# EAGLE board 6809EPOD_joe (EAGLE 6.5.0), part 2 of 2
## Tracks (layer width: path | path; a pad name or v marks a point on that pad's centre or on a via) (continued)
N$122  (via drill 0.2) (continued)
  Top 0.152: v44.73,49.61 44.27,50.06 40.92,50.06 40.16,50.82 32.54,50.82 31.62,51.74 18.21,51.74 17.91,51.44 17.91,50.52 17.45,50.06 12.57,50.06 12.27,49.76 12.27,49.15 v11.66,48.54
  Bottom 0.152: U14.5 47.07,46.96 45.19,46.96 44.73,47.47 v44.73,49.61 | RS11.R4A 10.36,49 11.2,49 v11.66,48.54
N$123  (via drill 0.2)
  Top 0.152: v45.03,50.82 44.58,50.37 41.07,50.37 40.31,51.13 32.69,51.13 31.77,52.05 18.06,52.05 17.6,51.59 17.6,50.67 17.3,50.37 12.12,50.37 v11.51,49.76
  Bottom 0.152: 47.07,49.5 U14.7 47.07,49.55 45.8,49.55 45.49,49.86 45.49,50.37 v45.03,50.82 | RS11.R3A v11.51,49.76
N$124  (via drill 0.2)
  Top 0.152: U5.14 19.3,9.37 20.8,9.37 21.72,8.46 23.7,8.46 24.15,8 28.27,8 29.79,6.48 36.04,6.48 37.57,4.95 38.33,4.95 38.79,5.41 38.79,7.24 39.55,8 39.55,9.22 40.92,10.59 40.92,11.2 41.53,11.81 46.41,11.81 v47.02,12.42 | v49.61,27.51 v51.89,27.51
  Bottom 0.152: v47.02,12.42 47.02,13.49 49.61,16.08 49.61,19.89 49,20.5 49,21.41 49.61,22.02 v49.61,27.51 | v51.89,27.51 54.33,27.51 54.79,27.96 54.79,30.71 54.48,31.01 52.65,31.01 53.42,31.17 53.37,31.12 U2.12
N$125  (via drill 0.2)
  Top 0.152: v17.45,16.84 17.75,17.14 U5.8 19.13,17.14
  Bottom 0.152: U10.3 17.6,20.95 17.45,20.8 17.45,19.74 | v17.45,16.84 17.45,19.74 | U10.2 19.1,19.74 17.45,19.74
N$126  (via drill 0.2)
  Top 0.152: v17.45,22.17 18.06,21.56 20.8,21.56 22.02,22.78 v33.15,22.78 | U6.6 37.01,34.87 36.96,34.98 34.82,34.98 v33.76,33.91
  Bottom 0.152: U10.4 19.07,22.22 18.82,22.17 v17.45,22.17 | v33.15,22.78 33.76,23.39 v33.76,33.91
N$127
  Top 0.152: U5.13 19.1,10.74 17.91,10.74 17.6,11.05 17.6,14.25 17.91,14.55 19.05,14.55 U5.10
N$128  (via drill 0.2)
  Top 0.152: v20.8,24.92 21.72,24.92 22.63,24 28.42,24 v28.88,24.46
  Bottom 0.152: U10.6 19.15,24.74 19.28,24.92 v20.8,24.92 | v28.88,24.46 28.88,23.85 29.18,23.55 30.56,23.55 30.58,23.52 U9.5
N$129  (via drill 0.2)
  Top 0.152: v22.78,16.99 24.92,16.99 25.07,17.14 U5.7 | U5.12 19.2,12.12 v22.33,12.12 | v29.03,21.56 28.12,22.48 24.92,22.48 24,21.56 23.39,21.56 v22.48,20.65
  Bottom 0.152: 25.68,19.74 25.63,19.68 U10.13 25.25,19.89 22.48,19.89 | 22.48,19.89 22.78,19.58 v22.78,16.99 22.33,16.69 v22.33,12.12 | U9.4 30.2,22.38 30.15,22.22 30,22.22 30.1,22.33 29.18,22.33 29.03,22.17 v29.03,21.56 | 22.48,19.89 v22.48,20.65
N$130  (via drill 0.2)
  Top 0.152: v23.7,20.8 24.46,20.8 24.61,20.65 27.81,20.65 v28.88,19.58
  Bottom 0.152: v23.7,20.8 25.22,20.8 25.07,20.95 U10.12 | U9.2 30.53,19.58 v28.88,19.58 28.88,18.82 29.18,18.52 30.48,18.52 U9.1
N$131  (via drill 0.2)
  Top 0.152: v33.15,9.07 33.15,9.98 34.82,11.66 34.82,13.03 35.13,13.34 U7.4 | v33.15,21.41 v33.15,19.43
  Bottom 0.152: v33.15,19.43 31.77,20.8 31.01,20.8 30.4,20.95 U9.3 | v33.15,9.07 32.69,9.53 32.69,12.57 34.21,14.1 34.21,15.32 33.3,16.23 33.3,16.99 34.37,18.06 34.37,20.19 v33.15,21.41
N$132  (via drill 0.2)
  Top 0.152: U5.3 25.3,11.96 v27.05,11.96 | U7.6 36.7,15.88 36.65,15.77 35.28,15.77 34.21,14.71 v33.3,14.71
  Bottom 0.152: v27.05,11.96 27.66,12.57 27.66,16.38 28.27,16.99 30.1,16.99 32.38,14.71 v33.3,14.71
RS17_TGT_BA  (via drill 0.2)
  Top 0.152: v73.23,4.65 73.23,6.17 73.53,6.48 79.17,6.48 79.78,7.09 v84.05,7.09
  Bottom 0.152: U13_PIGGY.3 71.55,5.71 71.7,5.56 72.92,5.56 73.23,5.26 v73.23,4.65 | v84.05,7.09 84.35,7.39 84.35,14.71 TGT_HDR.6
RS17_TGT_BS  (via drill 0.2)
  Top 0.152: v72.47,11.96 72.47,11.51 72.77,11.2 77.19,11.2 77.95,11.96 81.76,11.96 83.13,13.34 TGT_HDR.5
  Bottom 0.152: U13_PIGGY.6 72.47,9.53 72.62,9.68 72.62,11.81 v72.47,11.96
SEL_ADDR_TO_TGT  (via drill 0.2)
  Top 0.152: J8.11 5.82,15.88 5.87,15.93 9.07,15.93 10.13,16.99 16.54,16.99 17.91,18.36 v21.41,18.36 | U3.6 25.22,34.21 v23.7,34.21
  Bottom 0.152: v21.41,18.36 20.65,19.13 20.65,21.56 22.33,23.24 22.33,25.38 24.92,27.96 24.92,33.6 24.31,34.21 v23.7,34.21
SEL_ADDR_TO_TGT'  (via drill 0.2)
  Top 0.152: U20.1 67.74,41.88 v67.74,40.62 | v66.98,29.18 66.37,29.79 66.37,34.67 v66.83,35.13 | U22.1 68.5,2.51 66.83,2.51 66.52,2.82 v66.52,3.43 | 25.32,35.59 25.38,35.59 | 25.32,35.59 U3.7 | v51.28,35.59 55.7,35.59 56.46,34.82 59.36,34.82 59.82,34.37 v60.43,34.37 | U7.12 30.63,12.12 | v45.49,16.84 44.88,16.84 44.58,17.14 39.7,17.14 39.24,17.6 39.24,18.67 38.79,19.13 36.5,19.13 35.28,17.91 35.28,16.54 34.21,15.47 32.84,15.47 32.54,15.16 32.54,14.25 32.23,13.95 29.03,13.95 28.73,13.64 28.73,12.12 | v49,17.6 50.52,17.6 50.82,17.3 50.82,14.71 51.13,14.4 52.65,14.4 53.57,15.32 55.4,15.32 55.7,15.62 55.7,16.38 56.62,17.3 58.75,17.3 59.82,18.36 59.82,19.89 60.27,20.34 64.24,20.34 65.15,21.26 66.22,21.26 66.67,21.72 v66.67,23.09 | 25.32,35.59 24,35.59 v23.39,36.2 22.48,35.28 22.48,27.81 23.39,26.9 27.05,26.9 v28.27,25.68 | v27.2,10.9 27.66,10.9 27.96,11.2 27.96,11.81 28.27,12.12 28.73,12.12 | U7.12 30.45,12.07 30.4,12.12 28.73,12.12 | 30.71,12.12 30.66,12.07 U7.12
  Bottom 0.152: U19.1 71.25,40.62 v67.74,40.62 66.83,39.7 v66.83,35.13 61.19,35.13 v60.43,34.37 | U21.1 69.93,29.18 v66.98,29.18 66.98,28.12 67.59,27.51 67.59,23.09 | 67.59,23.09 67.59,21.26 67.89,20.95 67.89,15.01 67.28,14.4 67.28,11.35 65.61,9.68 65.61,8.31 66.06,7.85 66.06,3.89 v66.52,3.43 | U13.11 23.7,47.62 23.24,47.17 23.24,41.99 24.31,40.92 24.31,37.11 v23.39,36.2 | U2.10 53.14,33.6 52.05,33.6 51.28,34.37 v51.28,35.59 | v45.49,16.84 45.8,17.14 U8.2 48.54,17.14 v49,17.6 | v66.67,23.09 67.59,23.09 | v28.27,25.68 28.27,19.89 27.96,19.58 27.96,17.91 25.53,15.47 25.53,11.51 26.14,10.9 v27.2,10.9
TGT_A0  (via drill 0.2)
  Top 0.152: TGT_HDR.8 81.81,19.58 79.02,19.58 77.34,21.26 v74.3,21.26 | U22.4 68.5,6.33 72.47,6.33 73.53,7.39 v73.99,7.39
  Bottom 0.152: v73.99,7.39 74.45,7.85 74.45,9.83 73.99,10.29 73.99,15.93 74.3,16.23 v74.3,21.26
TGT_A1  (via drill 0.2)
  Top 0.152: TGT_HDR.9 81.86,22.17 81.86,20.45 81.3,19.89 79.17,19.89 76.89,22.17 v74.3,22.17 | U22.7 68.5,10.13 69.88,10.13 70.03,9.98 70.03,8 70.48,7.54 72.92,7.54 v73.69,8.31
  Bottom 0.152: v73.69,8.31 74.14,8.76 74.14,9.68 73.69,10.13 73.69,16.08 73.99,16.38 73.99,20.65 73.69,20.95 73.69,21.56 v74.3,22.17
TGT_A2  (via drill 0.2)
  Top 0.152: v78.56,24.61 77.8,25.38 76.73,25.38 76.12,24.77 71.25,24.77 69.88,26.14 v65.15,26.14 | U22.9 62.41,11.35 v64.08,11.35
  Bottom 0.152: TGT_HDR.10 81.76,24.61 v78.56,24.61 | v64.08,11.35 65.15,11.35 65.46,11.66 65.46,12.57 65.15,12.88 65.15,15.32 65.46,15.62 65.46,18.82 65.91,19.28 65.91,21.11 65.15,21.87 v65.15,26.14
TGT_A3  (via drill 0.2)
  Top 0.152: v66.83,27.2 67.59,26.44 70.03,26.44 71.4,25.07 75.97,25.07 77.19,26.29 v77.95,26.29 | U22.12 62.41,7.54 v64.69,7.54
  Bottom 0.152: v64.69,7.54 64.69,10.13 65.76,11.2 65.76,12.73 65.46,13.03 65.46,15.16 65.76,15.47 65.76,18.67 66.22,19.13 66.22,21.26 65.46,22.02 65.46,23.55 65.76,23.85 66.83,23.85 67.28,24.31 67.28,26.75 v66.83,27.2 | v77.95,26.29 79.48,27.51 82.07,27.51 83.13,28.57 TGT_HDR.11
TGT_A4  (via drill 0.2)
  Top 0.152: TGT_HDR.12 83.13,31.17 82.07,30.1 82.07,25.07 81.61,24.61 79.93,24.61 78.72,25.83 78.72,26.59 78.26,27.05 71.7,27.05 71.25,26.59 70.33,26.59 v69.72,27.2
  Bottom 0.152: U21.4 69.98,32.99 71.25,32.99 71.55,32.69 71.55,28.57 71.25,28.27 70.18,28.27 69.72,27.81 v69.72,27.2
TGT_A5  (via drill 0.2)
  Top 0.152: TGT_HDR.13 81.76,32.23 81.76,25.22 81.46,24.92 80.09,24.92 79.02,25.98 79.02,26.75 78.41,27.36 v70.79,27.36
  Bottom 0.152: U21.7 69.98,36.8 71.55,36.8 71.86,36.5 71.86,28.42 v70.79,27.36
TGT_A6  (via drill 0.2)
  Top 0.152: v78.26,37.57 81.91,37.57 83.13,36.35 83.13,36.25 TGT_HDR.14
  Bottom 0.152: U21.9 76.17,38.18 77.65,38.18 v78.26,37.57
TGT_A7
  Bottom 0.152: U21.12 75.87,34.06 78.56,34.06 79.48,34.98 79.48,37.11 79.93,37.57 81.91,37.57 83.13,38.79 TGT_HDR.15
TGT_A8
  Top 0.152: U20.4 68.55,45.8 76.28,45.8 77.04,45.03 81.46,45.03 81.91,44.58 81.91,42.6 83.13,41.38 83.13,41.33 TGT_HDR.16
TGT_A9  (via drill 0.2)
  Top 0.152: U20.7 68.5,49.55 68.5,49.61 69.88,49.61 70.33,49.15 70.33,46.56 70.79,46.1 77.95,46.1 v79.32,47.47
  Bottom 0.152: TGT_HDR.17 81.91,45.09 81.91,46.86 81.3,47.47 v79.32,47.47
TGT_A10
  Top 0.152: TGT_HDR.18 81.91,47.62 80.24,47.62 78.41,49.45 73.23,49.45 71.25,51.44 65.76,51.44 65,50.67 62.36,50.67 U20.9
TGT_A11  (via drill 0.2)
  Top 0.152: TGT_HDR.19 82.02,50.06 79.93,50.06 78.87,51.13 72.92,51.13 v72.62,51.44 | U20.12 62.36,47.02 v64.54,47.02
  Bottom 0.152: v64.54,47.02 60.58,47.02 60.27,47.32 60.27,50.06 61.65,51.44 v72.62,51.44
TGT_A12
  Bottom 0.152: U19.4 71.25,44.42 73.38,44.42 73.99,45.03 73.99,48.39 73.53,48.84 73.53,50.67 73.99,51.13 78.87,51.13 79.78,50.22 82.07,50.22 83.13,51.28 83.13,51.44 TGT_HDR.20
TGT_A13
  Bottom 0.152: U19.7 71.25,48.23 72.62,48.23 73.23,48.84 73.23,50.82 73.84,51.44 TGT_HDR.21
TGT_A14
  Bottom 0.152: U19.9 77.44,49.61 78.87,49.61 79.63,48.84 80.7,48.84 TGT_HDR.22
TGT_A15
  Bottom 0.152: U19.12 77.44,45.8 78.87,45.8 79.48,46.41 80.59,46.41 TGT_HDR.23
TGT_AVMA  (via drill 0.2)
  Top 0.152: v73.08,19.13 78.11,19.13 79.93,17.3 81.3,17.3 81.76,16.84 81.76,14.4 80.7,13.34 80.64,13.23 TGT_HDR.36
  Bottom 0.152: U11.5 71.3,19.13 v73.08,19.13
TGT_BUSY  (via drill 0.2)
  Top 0.152: v72.92,23.7 73.69,22.94 76.58,22.94 78.56,20.95 TGT_HDR.33 80.7,20.95
  Bottom 0.152: U11.7 71.25,21.56 72.62,21.56 72.92,21.87 v72.92,23.7
TGT_D0
  Top 0.152: U12.2 73,29.18 77.04,29.18 79.32,26.9 79.32,26.29 79.63,25.98 80.59,25.98 TGT_HDR.31
TGT_D1
  Top 0.152: U12.3 73.05,30.56 76.12,30.56 78.11,28.57 TGT_HDR.30
TGT_D2
  Top 0.152: U12.4 73,31.77 76.12,31.77 76.89,31.01 80.54,31.01 TGT_HDR.29
TGT_D3
  Top 0.152: U12.5 73,32.99 75.51,32.99 76.58,31.93 78.72,31.93 80.54,33.76 TGT_HDR.28
TGT_D4
  Top 0.152: U12.6 73.05,34.37 74.45,34.37 74.91,33.91 78.41,33.91 80.7,36.2 TGT_HDR.27
TGT_D5
  Top 0.152: U12.7 73,35.59 74.45,35.59 77.65,38.79 80.59,38.79 TGT_HDR.26
TGT_D6
  Top 0.152: U12.8 73,36.8 74.45,36.8 75.21,37.57 75.21,39.09 77.34,41.22 80.59,41.22 TGT_HDR.25
TGT_D7
  Top 0.152: U12.9 73.05,38.18 74.6,38.18 74.91,38.48 74.91,39.24 79.48,43.81 TGT_HDR.24 80.7,43.81
TGT_D_DIR  (via drill 0.2)
  Top 0.152: 72.8,28.09 72.77,28.12 v76.89,28.12 | 72.8,28.09 U12.1 | 72.8,28.09 68.99,28.09 68.66,28.42 68.66,29.64 68.2,30.1 v67.59,30.1 | v61.04,30.56 61.04,29.49 59.05,27.51 56.46,27.51 55.7,28.27 53.72,28.27 52.05,26.59 v48.84,26.59 | v48.84,24.77 46.86,24.77 44.42,22.33 40.92,22.33 40.46,22.78 36.8,22.78 35.59,21.56 v34.98,21.56 | v33.76,12.12 32.54,13.34 U7.11
  Bottom 0.152: U11.14 75.84,16.51 75.51,16.84 75.51,26.75 v76.89,28.12 | v61.04,30.56 61.04,31.32 61.34,31.62 66.67,31.62 67.59,30.71 v67.59,30.1 | v48.84,24.77 v48.84,26.59 | v34.98,21.56 35.28,21.26 35.28,13.64 v33.76,12.12
TGT_D_EN*  (via drill 0.2)
  Top 0.152: v49,22.63 52.05,22.63 52.5,23.09 v52.5,24.61 | v60.12,27.2 60.12,28.12 61.19,29.18 62.71,29.18 62.74,29.21 U12.19
  Bottom 0.152: U8.6 47.19,22.33 48.69,22.33 v49,22.63 | v52.5,24.61 53.11,25.22 55.24,25.22 56.01,25.98 56.01,26.44 56.77,27.2 v60.12,27.2
TGT_FIRQ*  (via drill 0.2)
  Top 0.152: v66.06,22.33 62.43,22.33 U17.9 62.2,22.22 62.1,22.33 v60.73,22.33 | v66.67,12.12 69.27,12.12 69.88,12.73 71.09,12.73 71.4,12.42 71.4,11.51 72.31,10.59 79.17,10.59 80.09,9.68 82.07,9.68 TGT_HDR.4 | v21.72,48.84 v28.12,48.84 | v33.76,47.02 40,47.02 40.62,47.62 44.58,47.62 45.03,47.17 v49.15,47.17 | v50.67,31.32 55.24,31.32 55.7,30.86 55.7,30.25 56.31,29.64 v59.66,29.64
  Bottom 0.152: v66.06,22.33 67.59,20.8 67.59,15.16 66.67,14.25 v66.67,12.12 | U13.5 19.2,48.84 v21.72,48.84 | v28.12,48.84 28.88,48.08 28.88,47.32 29.79,46.41 33.15,46.41 v33.76,47.02 | v49.15,47.17 49.61,46.71 49.61,37.57 50.06,37.11 50.06,31.93 v50.67,31.32 | v59.66,29.64 64.69,29.64 65.3,29.03 65.3,27.51 64.54,26.75 64.54,25.38 61.49,22.33 v60.73,22.33
TGT_HALT*  (via drill 0.2)
  Top 0.152: 70.18,15.77 71.09,14.86 v75.06,14.86 | 70.18,15.77 68.58,15.77 U17.1 68.48,15.77 70.18,15.77 | v21.72,43.81 21.72,45.95 22.17,46.41 v28.12,46.41 | 70.18,15.77 70.18,24.46 69.42,25.22 66.67,25.22 v66.06,24.61 | v65.15,37.26 65.15,35.43 65.76,34.82 65.76,31.47 v65.15,30.86 | v34.52,47.62 40.16,47.62 40.46,47.93 44.58,47.93 45.03,48.39 52.65,48.39 56.16,44.88 59.66,44.88 60.73,43.81 60.73,41.22 61.04,40.92 v65.15,40.92
  Bottom 0.152: TGT_HDR.40 80.59,3.12 80.39,2.97 79.78,2.36 75.06,2.36 74.6,2.82 74.6,5.26 75.06,5.71 v75.06,14.86 | U13.1 v21.72,43.81 | v66.06,24.61 66.06,29.95 v65.15,30.86 | v65.15,40.92 v65.15,37.26 | v28.12,46.41 28.12,42.44 28.57,41.99 33.45,41.99 34.06,42.6 34.06,44.58 34.52,45.03 v34.52,47.62
TGT_IRQ*  (via drill 0.2)
  Top 0.152: TGT_HDR.3 84.35,9.42 84.35,14.1 83.9,14.55 82.53,14.55 81.91,13.95 81.91,12.73 81.46,12.27 78.11,12.27 76.89,13.49 73.84,13.49 73.38,13.95 70.18,13.95 69.57,14.55 67.28,14.55 66.37,15.47 v66.37,15.93 | 62.38,18.36 U17.12 62.43,18.36 | 62.43,18.36 v66.37,18.36 | v28.12,47.62 v21.72,47.62 | v36.8,46.1 v33.76,46.1 | v35.89,41.22 36.2,40.92 39.7,40.92 40.46,40.16 43.66,40.16 45.03,41.53 v49,41.53 | v50.22,14.86 50.98,14.1 52.81,14.1 53.72,15.01 55.55,15.01 56.01,15.47 56.01,16.23 56.77,16.99 58.9,16.99 60.27,18.36 62.43,18.36
  Bottom 0.152: v66.37,18.36 v66.37,15.93 | U13.3 19.2,46.41 21.26,46.41 21.72,46.86 v21.72,47.62 | v33.76,46.1 29.64,46.1 v28.12,47.62 | v35.89,41.22 35.89,44.42 36.8,45.34 v36.8,46.1 | v49,41.53 49,37.72 49.76,36.96 49.76,29.49 51.13,28.12 51.13,26.14 50.52,25.53 50.52,15.16 v50.22,14.86
TGT_LIC  (via drill 0.2)
  Top 0.152: v73.38,16.69 77.19,16.69 77.8,16.08 77.8,13.49 78.11,13.18 v78.87,13.18
  Bottom 0.152: U11.3 71.4,16.69 v73.38,16.69 | v78.87,13.18 79.17,12.88 79.17,9.83 79.48,9.53 79.48,8.61 79.78,8.31 80.54,8.31 TGT_HDR.38
TGT_NMI*  (via drill 0.2)
  Top 0.152: v49.91,47.78 52.81,47.78 56.01,44.58 56.01,43.05 56.31,42.75 59.82,42.75 60.43,42.14 60.43,41.07 60.88,40.62 64.08,40.62 64.69,40 64.69,38.63 65,38.33 67.74,38.33 70.48,41.07 v73.38,41.07 | v74.3,5.87 74.6,6.17 79.32,6.17 79.93,6.78 82.07,6.78 83.13,5.71 TGT_HDR.2 | v50.67,29.95 47.62,26.9 v44.42,26.9 | v38.02,8.46 36.65,7.09 35.13,7.09 33.91,8.31 32.84,8.31 32.38,8.76 32.38,9.68 34.52,11.81 34.52,14.1 34.98,14.55 36.65,14.55 36.7,14.61 U7.5
  Bottom 0.152: U14.6 47.12,48.39 49.3,48.39 v49.91,47.78 49.91,37.72 50.37,37.26 50.37,32.99 50.67,32.69 51.44,32.69 51.74,32.38 51.74,29.95 | v73.38,41.07 73.84,40.62 73.84,27.66 74.91,26.59 74.91,16.38 74.3,15.77 74.3,10.44 74.75,9.98 74.75,6.33 v74.3,5.87 | U2.13 53.19,29.95 51.74,29.95 | v50.67,29.95 51.74,29.95 | v44.42,26.9 44.42,25.83 45.03,25.22 45.03,24.61 44.73,24.31 44.73,20.95 43.36,19.58 41.07,19.58 40.77,19.28 40.77,13.34 39.39,11.96 38.48,11.96 38.02,11.51 v38.02,8.46
TGT_R/W
  Bottom 0.152: U11.13 77.39,17.91 76.12,17.91 75.82,18.21 75.82,23.24 76.12,23.55 80.59,23.55 TGT_HDR.32
TGT_RST*  (via drill 0.2)
  Top 0.152: TGT_HDR.37 80.59,10.9 72.47,10.9 71.7,11.66 71.7,12.42 72.01,12.73 72.77,12.73 73.99,11.51 76.28,11.51 76.58,11.81 76.58,12.57 76.28,12.88 73.53,12.88 73.08,13.34 69.88,13.34 69.27,13.95 65.3,13.95 64.69,14.55 56.62,14.55 55.85,13.79 v54.33,13.79 | J7.32 13.23,41.27 12.42,40.46 7.09,40.46 6.63,40 4.8,40 4.5,39.7 4.5,2.36 4.95,1.91 16.54,1.91 16.99,2.36 16.99,4.5 17.75,5.26 24.77,5.26 25.68,4.34 25.68,3.28 26.14,2.82 39.39,2.82 41.07,4.5 43.97,4.5 44.58,3.89 44.58,3.28 45.03,2.82 49.91,2.82 v50.22,3.12 | v73.84,23.7 78.11,23.7 v79.32,22.48
  Bottom 0.152: CR1.A 73.08,25.83 73.08,24.46 v73.84,23.7 | v79.32,22.48 79.32,15.32 79.78,14.86 79.78,14.25 79.48,13.95 79.48,11.96 TGT_HDR.37 80.7,10.74 | v50.22,3.12 50.22,7.24 50.67,7.7 50.67,8.46 51.74,9.53 51.74,11.81 52.05,12.12 52.05,13.49 52.35,13.79 v54.33,13.79
TGT_VCC
  Bottom 0.61: 68B09E.7 57.84,18.36 C9.1
  pour vcc (isolate 0.254): 56.52,17.78 56.52,26.67 57.15,27.3 84.45,27.3 84.45,17.14 57.15,17.14
VCC  (via drill 0.2)
  Top 0.152: U22.3 68.45,5.1 v66.98,5.1 | U22.6 68.45,8.92 v66.83,8.92 | U22.10 62.51,9.98 v64.08,9.98 | U22.13 62.36,6.33 v64.08,6.33 | U20.6 68.45,48.23 v65.46,48.23 | U20.10 62.41,49.45 63.63,49.45 63.93,49.15 63.93,48.54 64.24,48.23 v65.46,48.23 | U20.13 62.41,45.64 65,45.64 65.46,46.1 v65.46,48.23 | U20.3 68.35,44.58 v66.52,44.58 | U6.13 32.23,29.79 32.38,29.64 32.38,28.73 | U6.1 37.01,28.52 36.96,28.73 32.38,28.73 | 28.73,28.57 31.32,28.73 32.38,28.73 | U6.4 37.08,32.38 36.5,32.38 36.35,32.23 v35.43,32.23 | v27.96,33.6 U6.10
  Top 0.406: U22.16 62.36,2.51 v63.93,2.51 | U17.14 62.56,15.88 62.1,15.77 v60.73,15.77 | U12.20 63.17,27.96 v64.54,27.96 | U20.16 62.41,41.99 v64.08,41.99 | U4.20 29.82,50.82 v31.47,50.82 | U3.16 19.18,27.96 v20.8,27.96 | U6.14 30.94,28.57 28.73,28.57 v28.12,29.18 | 30.71,9.53 U7.14 28.27,9.53 v27.81,9.07 | U5.4 v26.9,13.34 | C10.1 71.83,47.5 71.86,47.47 72.77,47.47 v73.23,47.02 | C4.1 76.86,34.8 76.89,34.82 v78.11,34.82 | C3.1 71.65,16.28 71.7,16.23 72.62,16.23 v73.08,15.77 | C17.1 72.47,8.76 72.92,9.22 v73.53,9.22 | R19.2 31.95,7.54 v33.15,7.54 | C8.1 21.26,4.27 v21.26,3.43 | C16.1 51.46,9.65 51.28,9.68 45.95,9.68 v45.49,9.53 | C18.1 52.81,43.16 v52.81,41.02
  Top 0.508: C1.+ 77.5,8.88 77.5,9.68 v75.82,9.68
  Bottom 0.152: U21.3 69.93,31.77 v68.2,31.77 | U21.6 69.93,35.59 v68.2,35.59 | U21.10 75.97,36.96 74.75,36.96 74.45,36.65 74.45,33.3 74.75,32.99 | U21.13 76.07,32.99 74.75,32.99 | U19.3 71.25,43.2 v73.23,43.2 | U19.13 77.34,44.42 v75.51,44.42 | U19.6 71.25,47.02 v73.23,47.02 | U19.10 77.34,48.23 v75.51,48.23 | 74.75,32.99 v78.11,32.99 | U13_PIGGY.14 75.62,3.17 75.36,3.43 75.36,9.22 v75.82,9.68
  Bottom 0.406: U16.20 29.87,3.89 v27.51,3.89 | U13_PIGGY.14 77.32,3.12 | U11.16 78.11,13.95 78.56,13.95 v79.17,14.55 | U21.16 76.12,29.18 77.5,29.18 v78.11,29.79 | U19.16 78.11,40.64 v78.11,39.7 | U14.16 53.26,41.83 53.19,41.91 52.65,41.91 52.58,41.83 52.81,41.83 v52.81,41.02 | U1.4 47.12,6.33 45.64,6.33 45.49,6.48 v45.49,7.54 47.17,7.54 U1.5 | U10.14 25.25,18.52 v23.7,18.52 | U2.14 53.24,28.6 53.72,28.57 v51.74,28.57 | U13.14 25.68,43.66 v25.68,42.9 | U15.20 29.77,29.18 v28.12,29.18 | U9.14 36.78,18.36 v38.33,18.36 | U8.14 52.5,15.88 v52.5,15.01 | C21.1 61.7,48.23 v65.46,48.23 67.84,48.23 C7.1 | C6.1 46.86,39.62 47.17,39.39 v46.1,39.39 | v68.2,35.59 67.89,35.89 67.89,36.65 C5.1 | C14.1 36.8,32.23 v35.43,32.23 | C11.1 36.83,10.62 36.35,10.13 v34.52,10.13 | C20.1 69.09,9.37 67.28,9.37 v66.83,8.92 | C19.1 61.8,12.85 61.8,14.71 v60.73,15.77 | C15.1 36.96,50.85 v36.96,49.91
  Bottom 0.508: C2.+ 31.47,48.78 v31.47,50.82
  pour vcc (isolate 0.254, rank 2): 0.64,53.34 1.27,53.98 31.75,53.98 32.38,53.34 32.38,52.07 33.02,51.44 40,51.44 40.64,52.07 40.64,53.34 41.27,53.98 69.85,53.98 71.12,52.7 83.82,52.7 84.45,52.07 84.45,2.54 83.82,1.91 71.12,1.91 69.85,0.64 1.27,0.64 0.64,1.27

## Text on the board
Top: 1
gnd: 2
vcc: 3
Bottom: 4
tPlace: TOP OF MAIN BOARD | 6809E POD | 2009 | Clone by Joe Britt | EM-189 | 1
